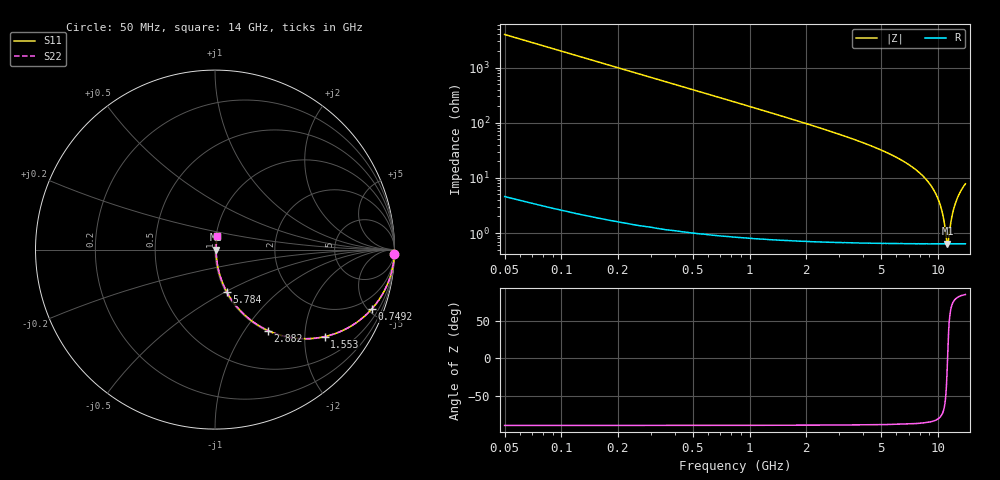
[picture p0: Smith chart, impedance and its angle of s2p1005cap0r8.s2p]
!	AVX	Thin	Film	Operation
!	Date:	March 2012
!	Description: Ultra-Miniature 01005 Size ACCU - P® Thin Film RF / Microwave Capacitor
!	Part Number:  C005YK0R8ABSTR
!	Serial	Measurements
#	MHz	S	db	R	50
!	S11	S21	S12	S22
!	dB	Phase	dB	Phase	dB	Phase	dB	Phase
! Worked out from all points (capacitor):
!   400 points, 50 MHz to 14 GHz, reference 50 ohm
!   read as one part in series: C = 800 fF near 119.9 MHz
!   lowest |Z| = 638 mohm at 11.24 GHz (marker M1)
!   series resonance near 11.25 GHz, so ESL is about 250 pH
!   S11 on the Smith chart (normalised r, x): 50 MHz: 1, -80; 749.2 MHz: 1.02, -5.29; 1.553 GHz: 1.01, -2.51; 2.882 GHz: 1.01, -1.29; 5.784 GHz: 1.01, -0.51; 14 GHz: 1.01, +0.16
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50  -0.00 -1.4  -32.00 88.5  -32.00 88.5  -0.00 -1.4
84.962  -0.01 -2.4  -27.40 87.5  -27.40 87.5  -0.01 -2.4
119.925  -0.02 -3.5  -24.41 86.5  -24.41 86.5  -0.02 -3.5
259.774  -0.07 -7.4  -17.75 82.5  -17.75 82.5  -0.07 -7.4
469.549  -0.24 -13.3  -12.77 76.6  -12.77 76.6  -0.24 -13.3
749.248  -0.59 -20.7  -9.03 69.1  -9.03 69.1  -0.59 -20.7
1553.383  -2.16 -38.4  -4.14 51.3  -4.14 51.3  -2.16 -38.4
2392.481  -4.16 -51.2  -2.16 38.3  -2.16 38.3  -4.16 -51.2
2881.955  -5.36 -56.8  -1.55 32.6  -1.55 32.6  -5.36 -56.8
4700  -9.68 -69.8  -0.55 19.1  -0.55 19.1  -9.68 -69.8
5783.835  -12.25 -74.4  -0.32 14.1  -0.32 14.1  -12.25 -74.4
7042.481  -15.47 -78.2  -0.18 9.7  -0.18 9.7  -15.47 -78.2
9350  -23.66 -80.7  -0.07 3.7  -0.07 3.7  -23.66 -80.7
9979.323  -27.38 -79.1  -0.06 2.4  -0.06 2.4  -27.38 -79.1
10468.8  -31.64 -74.6  -0.06 1.5  -0.06 1.5  -31.64 -74.6
10783.46  -35.76 -66.3  -0.06 0.9  -0.06 0.9  -35.76 -66.3
11237.97  -43.94 -4.5  -0.06 0.0  -0.06 0.0  -43.94 -4.5
11342.86  -43.21 23.4  -0.06 -0.2  -0.06 -0.2  -43.21 23.4
11692.48  -36.57 64.0  -0.06 -0.8  -0.06 -0.8  -36.57 64.0
12042.1  -32.17 73.7  -0.06 -1.4  -0.06 -1.4  -32.17 73.7
12531.58  -28.32 78.3  -0.06 -2.2  -0.06 -2.2  -28.32 78.3
14000  -22.23 80.9  -0.08 -4.4  -0.08 -4.4  -22.23 80.9
